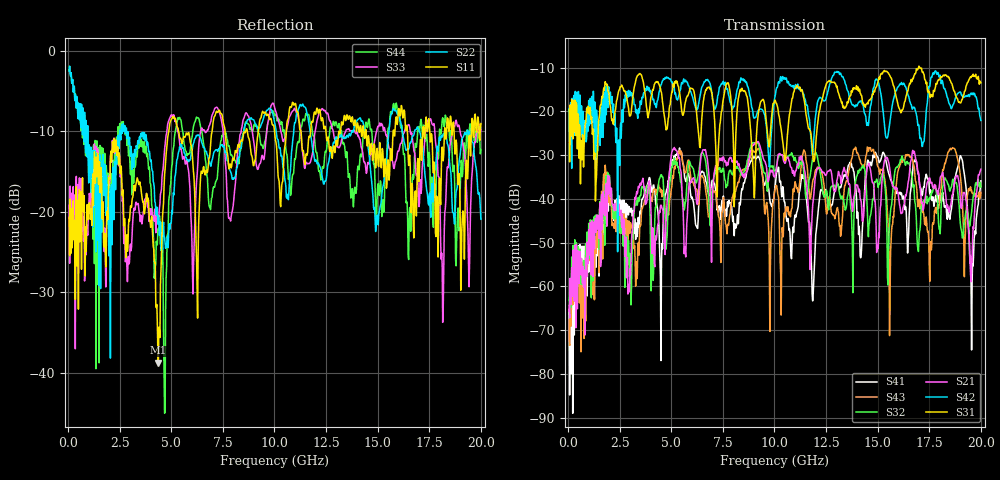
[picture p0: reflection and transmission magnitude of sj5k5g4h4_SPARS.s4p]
! FILE: E:\users\goganessyan\GBX_Backplane\FR408_backplane\1m_INBOUND_NEXT\sj5k5g4h4_SPARS.s4p
# MHZ S RI R 50.00
! FREQ  S11  S12  S13  S14
!  S21  S22  S23  S24
!  S31  S32  S33  S34
!  S41  S42  S43  S44
!  REAL  IMAG  REAL  IMAG  REAL  IMAG  REAL  IMAG
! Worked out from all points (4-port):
!   799 points, 50 MHz to 20 GHz, reference 50 ohm
!   strongest paths, dB at 50 MHz, 5.025 GHz, 10.03 GHz, 15.03 GHz, 20 GHz:
!     S31: -19.6, -15.6, -17.4, -13.2, -13.5
!     S42: -19.4, -13.3, -16.6, -13.1, -22.1
!     S21: -64.4, -29.3, -34.9, -51.4, -33.2
!     S32: -63.3, -32.6, -33.4, -37.4, -37.3
!     S43: -67.7, -37.3, -37.9, -32.7, -38.5
!     S41: -65.3, -32.3, -37.2, -30.6, -35.9
!   lowest |S11| = -38.8 dB at 4.375 GHz (marker M1), VSWR 1.02, Z = 50.3 + j1.13 ohm
!   |S11| at or under -10 dB: start of sweep to 4.877 GHz; 5.354 GHz to 6.977 GHz (1.622 GHz wide, 26.3 % of centre); 14.43 GHz to 15.75 GHz (1.314 GHz wide, 8.71 % of centre)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
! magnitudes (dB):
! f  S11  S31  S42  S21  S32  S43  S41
! 50 MHz  -20.7  -19.6  -19.4  -64.4  -63.3  -67.7  -65.3
! 4.375 GHz  -38.8  -13.5  -16.7  -45.8  -36.8  -36.7  -44.3
! 5.075 GHz  -8.1  -14.6  -14.2  -28.7  -31.4  -34.7  -31.1
! 11.88 GHz  -8.6  -30.9  -28.4  -40.5  -30.4  -35.5  -61.7
! 13.7 GHz  -8.7  -16.3  -17.8  -39.7  -42.3  -31.6  -31.9
! 19.55 GHz  -9.2  -11.9  -15.9  -55.7  -43.0  -38.0  -74.5
! 20 GHz  -9.0  -13.5  -22.1  -33.2  -37.3  -38.5  -35.9
